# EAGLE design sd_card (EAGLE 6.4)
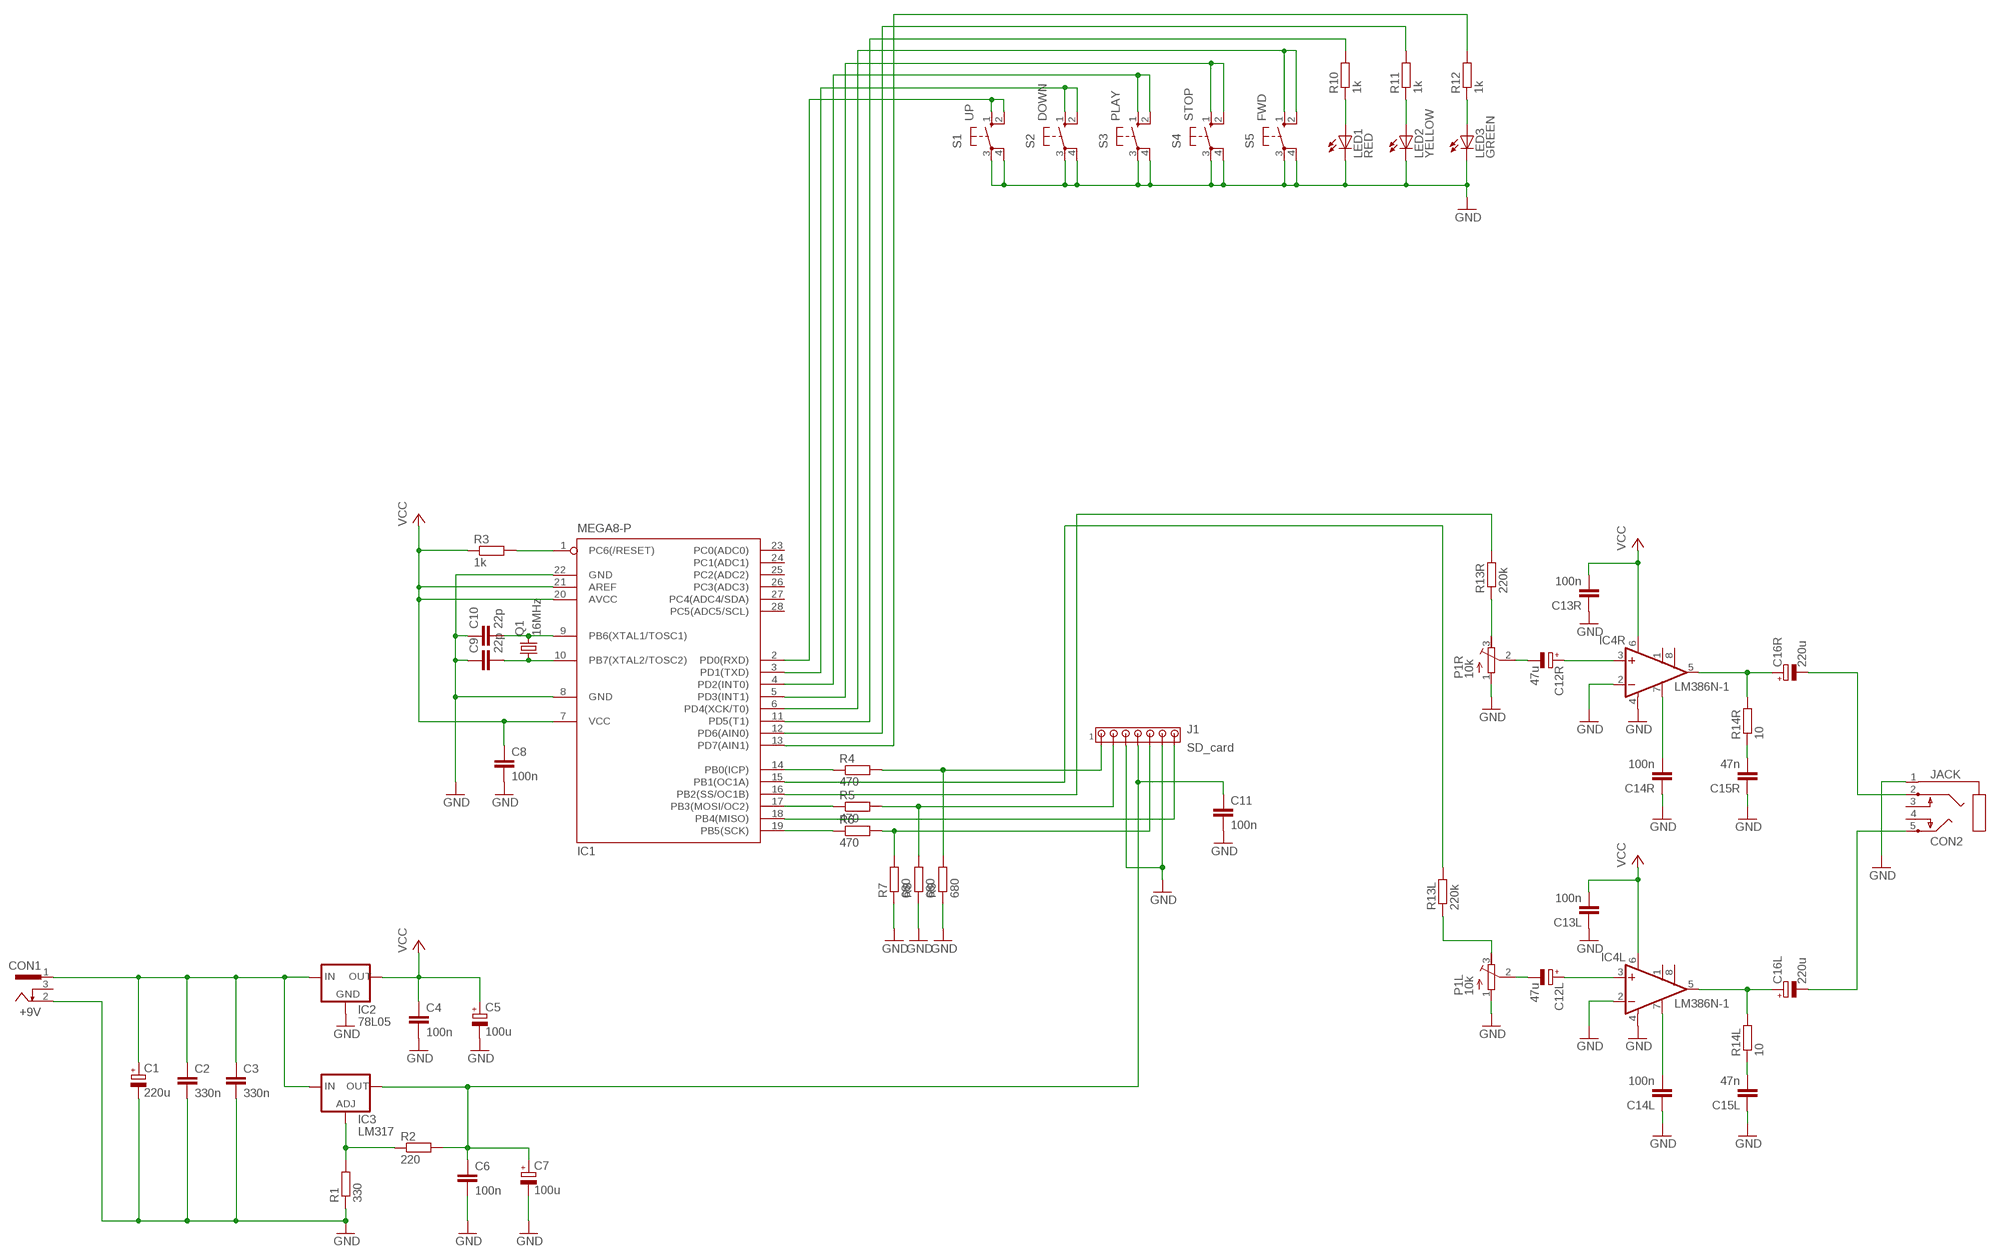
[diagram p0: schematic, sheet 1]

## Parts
C1  220u  CPOL-EUE5-8.5  [E5-8,5]
C2  330n  C-EU025-025X050  [C025-025X050]
C3  330n  C-EU025-025X050  [C025-025X050]
C4  100n  C-EU025-025X050  [C025-025X050]
C5  100u  CPOL-EUE2.5-5  [E2,5-5]
C6  100n  C-EU025-025X050  [C025-025X050]
C7  100u  CPOL-EUE2.5-5  [E2,5-5]
C8  100n  C-EU025-025X050  [C025-025X050]
C9  22p  C-EU025-025X050  [C025-025X050]
C10  22p  C-EU025-025X050  [C025-025X050]
C11  100n  C-EU025-025X050  [C025-025X050]
C12L  47u  CPOL-EUE2.5-5  [E2,5-5]
C12R  47u  CPOL-EUE2.5-5  [E2,5-5]
C13L  100n  C-EU025-025X050  [C025-025X050]
C13R  100n  C-EU025-025X050  [C025-025X050]
C14L  100n  C-EU025-025X050  [C025-025X050]
C14R  100n  C-EU025-025X050  [C025-025X050]
C15L  47n  C-EU025-025X050  [C025-025X050]
C15R  47n  C-EU025-025X050  [C025-025X050]
C16L  220u  CPOL-EUE5-4  [E5-4]
C16R  220u  CPOL-EUE5-4  [E5-4]
CON1  +9V  733980-62  [733980-62]
CON2  JACK  [JACK]
IC1  MEGA8-P  [DIL28-3]
IC2  78L05  78XXL  [78XXL]
IC3  LM317  LM317TL  [317TL]
IC4L  LM386N-1  [DIL08]
IC4R  LM386N-1  [DIL08]
J1  SD_card  MTA07-100  [10X07MTA]
LED1  RED  LED5MM  [LED5MM]
LED2  YELLOW  LED5MM  [LED5MM]
LED3  GREEN  LED5MM  [LED5MM]
P1L  10k  TRIM  [TRIM]
P1R  10k  TRIM  [TRIM]
Q1  16MHz  CRYSTALHC49S  [HC49/S]
R1  330  R-EU_0207/10  [0207/10]
R2  220  R-EU_0207/2V  [0207/2V]
R3  1k  R-EU_0207/10  [0207/10]
R4  470  R-EU_0207/10  [0207/10]
R5  470  R-EU_0207/10  [0207/10]
R6  470  R-EU_0207/10  [0207/10]
R7  680  R-EU_0207/10  [0207/10]
R8  680  R-EU_0207/10  [0207/10]
R9  680  R-EU_0207/10  [0207/10]
R10  1k  R-EU_0207/10  [0207/10]
R11  1k  R-EU_0207/10  [0207/10]
R12  1k  R-EU_0207/10  [0207/10]
R13L  220k  R-EU_0207/2V  [0207/2V]
R13R  220k  R-EU_0207/2V  [0207/2V]
R14L  10  R-EU_0207/10  [0207/10]
R14R  10  R-EU_0207/10  [0207/10]
S1  UP  10-XX  [B3F-10XX]
S2  DOWN  10-XX  [B3F-10XX]
S3  PLAY  10-XX  [B3F-10XX]
S4  STOP  10-XX  [B3F-10XX]
S5  FWD  10-XX  [B3F-10XX]

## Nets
GND: C1.- C2.2 C3.2 C4.2 C5.- C6.2 C7.- C8.2 C9.1 C10.1 C11.2 C13L.1 C13R.1 C14L.1 C14R.1 C15L.1 C15R.1 CON1.2 CON2.1 IC1.8(GND) IC1.22(GND) IC2.GND IC4L.2(-IN) IC4L.4(GND) IC4R.2(-IN) IC4R.4(GND) J1.3 J1.6 LED1.K(C) LED2.K(C) LED3.K(C) P1L.1 P1R.1 R1.1 R7.1 R8.1 R9.1 S1.3(P) S1.4(P1) S2.3(P) S2.4(P1) S3.3(P) S3.4(P1) S4.3(P) S4.4(P1) S5.3(P) S5.4(P1)
N$1: C1.+ C2.1 C3.1 CON1.1 IC2.IN IC3.3(IN)
N$2: IC3.1(ADJ) R1.2 R2.1
N$3: C6.1 C7.+ C11.1 IC3.2(OUT) J1.4 R2.2
N$4: IC1.14(PB0(ICP)) R4.1
N$5: C10.2 IC1.9(PB6(XTAL1/TOSC1)) Q1.2
N$6: C9.2 IC1.10(PB7(XTAL2/TOSC2)) Q1.1
N$7: IC1.17(PB3(MOSI/OC2)) R5.1
N$8: IC1.1(PC6(/RESET)) R3.2
N$9: C12R.+ IC4R.3(+IN)
N$10: IC1.19(PB5(SCK)) R6.1
N$11: J1.5 R6.2 R7.2
N$12: J1.2 R5.2 R8.2
N$13: J1.1 R4.2 R9.2
N$14: IC1.18(PB4(MISO)) J1.7
N$15: C16R.+ IC4R.5(OUT) R14R.2
N$16: C15R.2 R14R.1
N$17: C14R.2 IC4R.7(BYPASS)
N$18: C12R.- P1R.2
N$19: C16L.+ IC4L.5(OUT) R14L.2
N$20: C15L.2 R14L.1
N$21: C14L.2 IC4L.7(BYPASS)
N$22: C12L.+ IC4L.3(+IN)
N$23: LED3.A R12.1
N$24: LED2.A R11.1
N$25: LED1.A R10.1
N$26: IC1.2(PD0(RXD)) S1.1(S) S1.2(S1)
N$27: IC1.3(PD1(TXD)) S2.1(S) S2.2(S1)
N$28: IC1.4(PD2(INT0)) S3.1(S) S3.2(S1)
N$29: IC1.5(PD3(INT1)) S4.1(S) S4.2(S1)
N$30: IC1.6(PD4(XCK/T0)) S5.1(S) S5.2(S1)
N$31: IC1.11(PD5(T1)) R10.2
N$32: IC1.12(PD6(AIN0)) R11.2
N$33: IC1.13(PD7(AIN1)) R12.2
N$69: C12L.- P1L.2
N$70: C16R.- CON2.2
N$71: C16L.- CON2.5
N$73: IC1.16(PB2(SS/OC1B)) R13R.2
N$132: P1R.3 R13R.1
N$133: P1L.3 R13L.1
N$134: IC1.15(PB1(OC1A)) R13L.2
VCC: C4.1 C5.+ C8.1 C13L.2 C13R.2 IC1.7(VCC) IC1.20(AVCC) IC1.21(AREF) IC2.OUT IC4L.6(VS) IC4R.6(VS) R3.1
Unconnected: CON1.3 CON2.3 CON2.4 IC1.23(PC0(ADC0)) IC1.24(PC1(ADC1)) IC1.25(PC2(ADC2)) IC1.26(PC3(ADC3)) IC1.27(PC4(ADC4/SDA)) IC1.28(PC5(ADC5/SCL)) IC4L.1(GAIN) IC4L.8(GAIN) IC4R.1(GAIN) IC4R.8(GAIN)

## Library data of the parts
C1 C5 C7 C12L C12R C16L C16R = resistor:CPOL-EU: POLARIZED CAPACITOR, European symbol
C2-C4 C6 C8-C11 C13L C13R C14L C14R C15L C15R = rcl:C-EU: CAPACITOR, European symbol
CON1 = con-conrad:73398?: FEMALE PRINT CONNECTOR Niedervolt-Steckverbinder Distributor Conrad
CON2 = jack:JACK
IC1 = atmel:MEGA8-P: MICROCONTROLLER 8 Kbytes FLASH, 1 kbytes SRAM, 512 bytes EEPROM, USART, 4-channel 10 bit ADC, 2-channel 8 bit ADC Pin compatible with Atmega48, ATMega88, ATMega168 Source: avr.lbr; OC_FARNELL: unknown; OC_NEWARK: unknown
IC2 = v-reg:78XXL: VOLTAGE REGULATOR
IC3 = v-reg:LM317TL: VOLTAGE REGULATOR
IC4L IC4R = linear:LM386?-*: Low Voltage Audio Power Amplifier Source: http://cache.national.com/ds/LM/LM386.pdf
J1 = con-amp:MTA07-100: AMP connector
LED1-LED3 = led:LED: LED
P1L P1R = trim:TRIM
Q1 = crystal:CRYSTAL: CRYSTAL; OC_FARNELL: 1667008; OC_NEWARK: unknown
R1-R12 R13L R13R R14L R14R = rcl:R-EU_: RESISTOR, European symbol
S1-S5 = switch-omron:10-XX: OMRON SWITCH; MPN: B3F-1000; OC_FARNELL: 176432; OC_NEWARK: 36M3542

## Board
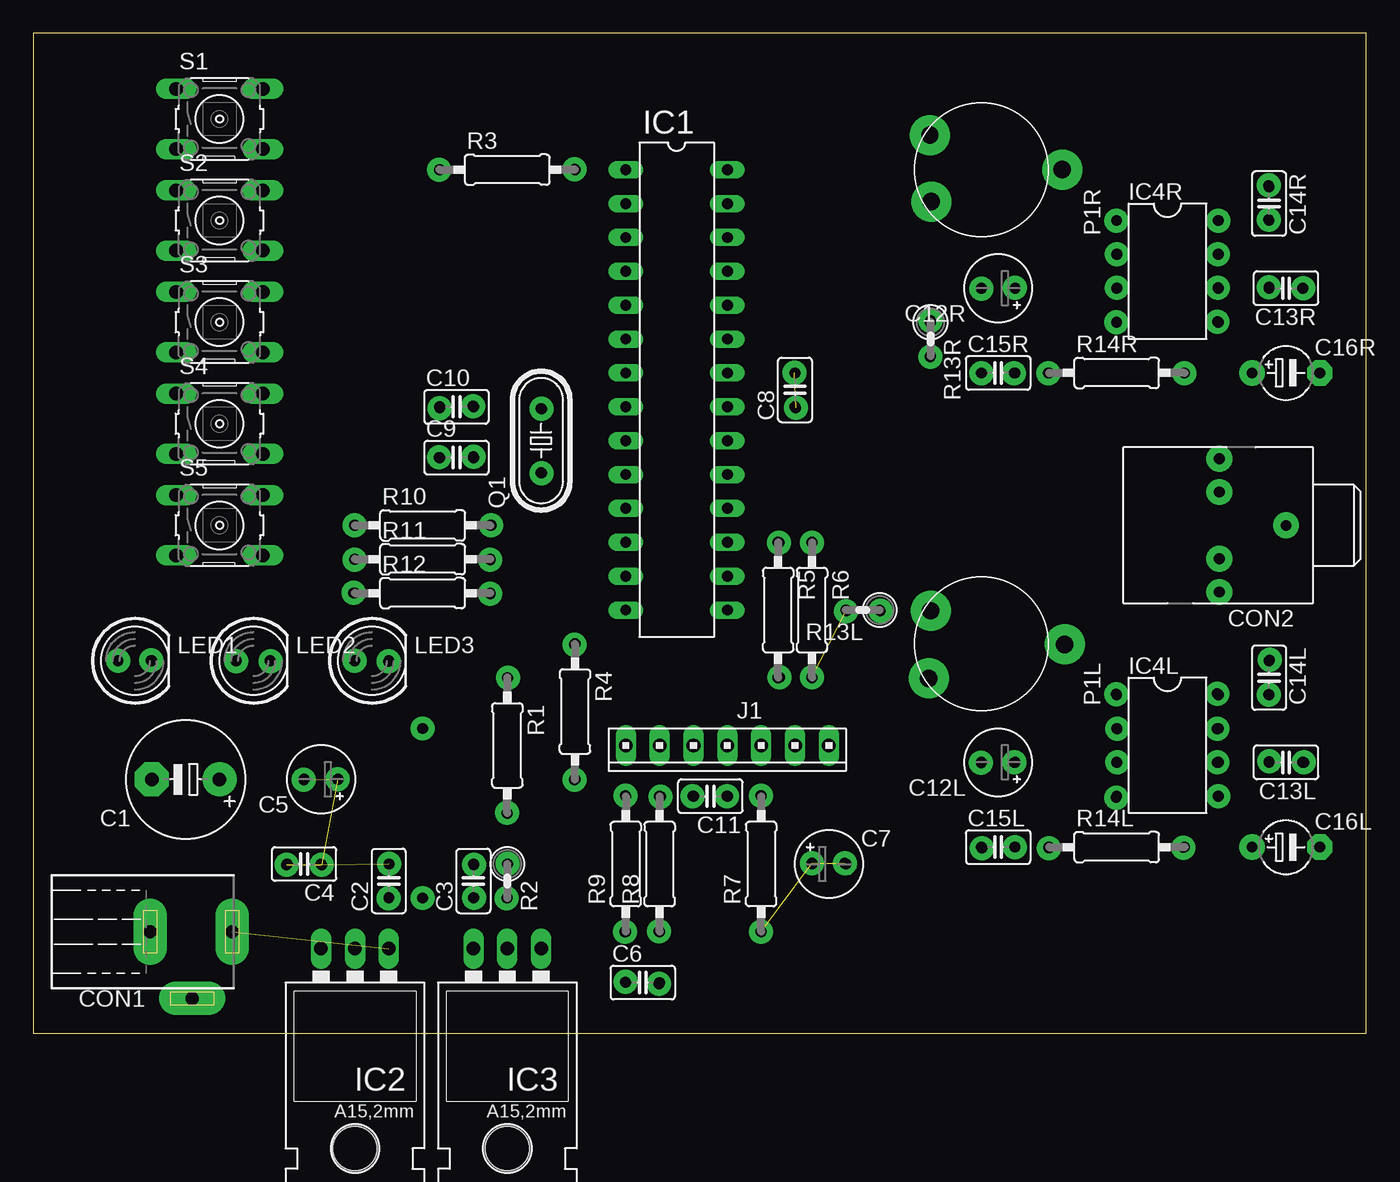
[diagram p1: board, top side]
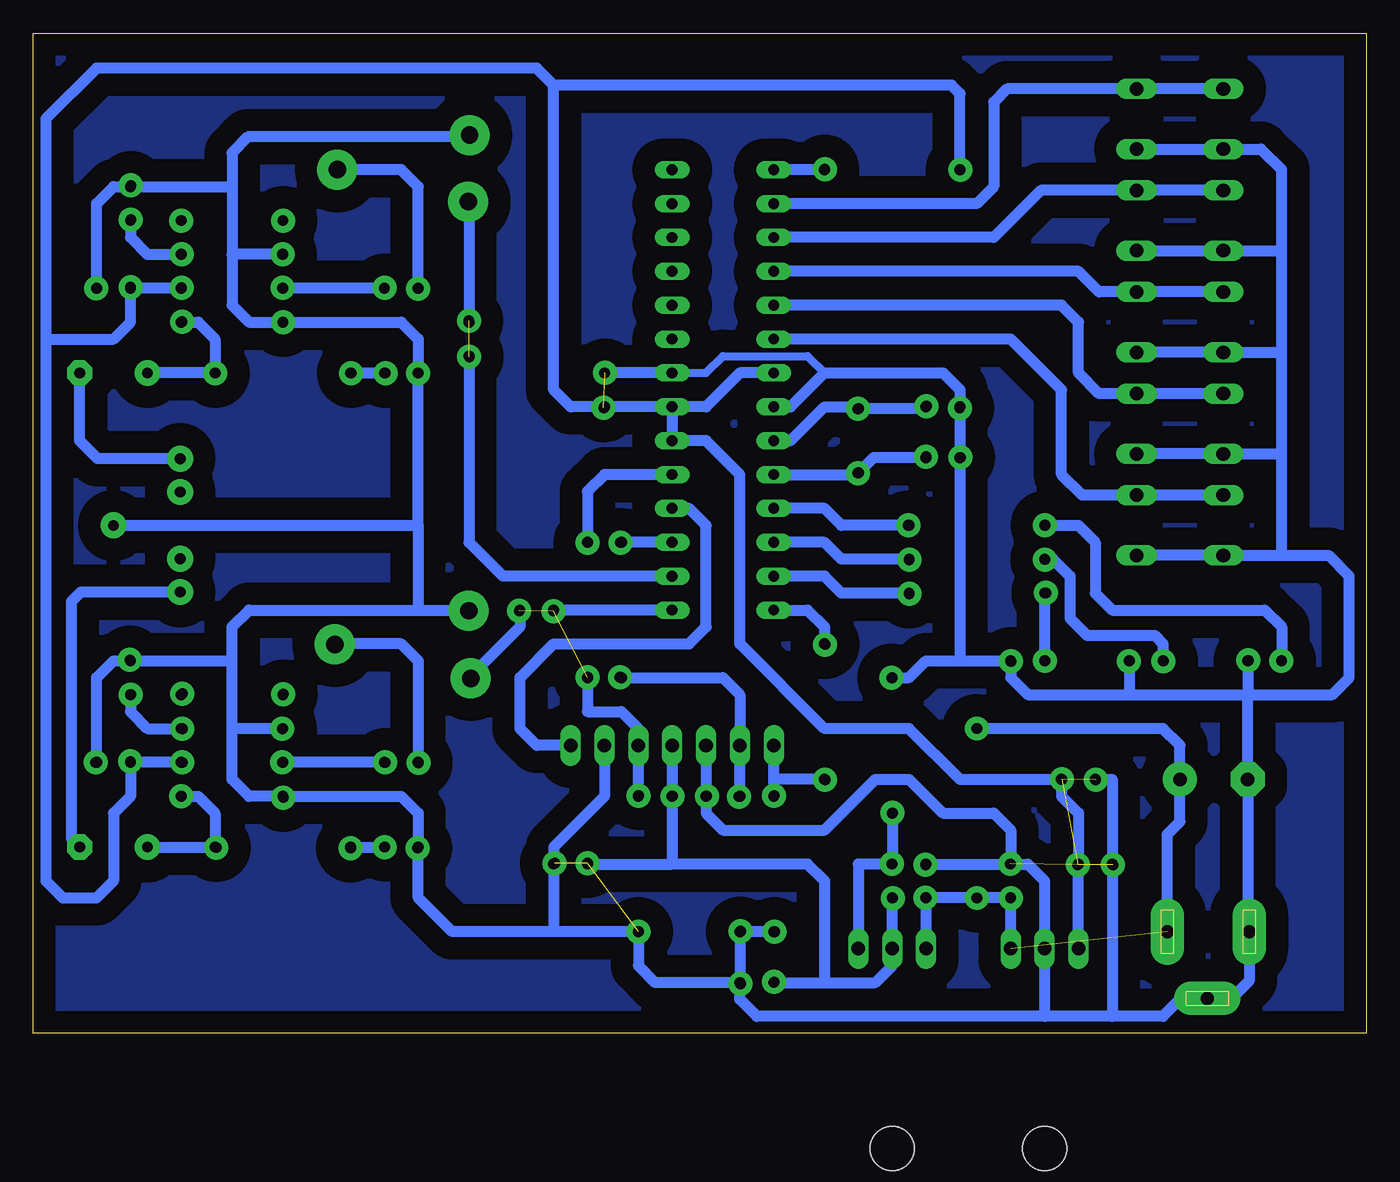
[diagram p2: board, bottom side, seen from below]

Size 100 x 75 mm. Coordinates in mm from the lower left corner, seen from the top.
Outline: 0,0 100,0 100,75 0,75 0,0
Copper layers (1*16): Top 0.035mm / dielectric 1.5mm / Bottom 0.035mm
Design rules "default": minimum track width 10mil, minimum drill 24mil, track to track 8mil, track to pad 8mil, pad to pad 8mil, via to via 8mil, smd to smd 8mil, copper to edge 40mil, drill to drill 8mil, minimum pad ring 10mil, minimum via ring 8mil, stop-mask expansion 4mil, vias tented up to drill 0mil, thermal gap 10mil

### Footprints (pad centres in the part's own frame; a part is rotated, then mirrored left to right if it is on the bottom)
E5-8,5 = drill 1.016 pad 2.54: + -2.54,0 | drill 1.016 pad 2.54 octagon: - 2.54,0
C025-025X050 = drill 0.813 octagon: 1 -1.27,0; 2 1.27,0
E2,5-5 = drill 0.813 pad 1.6: + -1.27,0 | drill 0.813 pad 1.6 octagon: - 1.27,0
E5-4 = drill 0.813 pad 1.905: + -2.54,0 | drill 0.813 pad 1.905 octagon: - 2.54,0
733980-62 = drill 1 pad 2.5 long: 1 0,8.57; 2 0,2.42; 3 5,5.57
JACK = drill 0.8 pad 1.93: 1 -5.08,0; 2 -0.08,-5; 3 -0.08,2.5; 4 -0.08,-2.5; 5 -0.08,5
DIL28-3 = drill 0.813 long: 1 -16.51,-3.81; 2 -13.97,-3.81; 3 -11.43,-3.81; 4 -8.89,-3.81; 5 -6.35,-3.81; 6 -3.81,-3.81; 7 -1.27,-3.81; 8 1.27,-3.81; 9 3.81,-3.81; 10 6.35,-3.81; 11 8.89,-3.81; 12 11.43,-3.81; 13 13.97,-3.81; 14 16.51,-3.81; 15 16.51,3.81; 16 13.97,3.81; 17 11.43,3.81; 18 8.89,3.81; 19 6.35,3.81; 20 3.81,3.81; 21 1.27,3.81; 22 -1.27,3.81; 23 -3.81,3.81; 24 -6.35,3.81; 25 -8.89,3.81; 26 -11.43,3.81; 27 -13.97,3.81; 28 -16.51,3.81
78XXL = drill 1.016 long: GND 0,-3.81; IN -2.54,-3.81; OUT 2.54,-3.81 | hole 3.302: 0,11.176
317TL = drill 1.016 long: 1 -2.54,-3.81; 2 0,-3.81; 3 2.54,-3.81 | hole 3.302: 0,11.176
DIL08 = drill 0.813 pad 1.27: 1 -3.81,-3.81; 2 -1.27,-3.81; 3 1.27,-3.81; 4 3.81,-3.81; 5 3.81,3.81; 6 1.27,3.81; 7 -1.27,3.81; 8 -3.81,3.81
10X07MTA = drill 1.016 long: 1 7.62,0; 2 5.08,0; 3 2.54,0; 4 0,0; 5 -2.54,0; 6 -5.08,0; 7 -7.62,0
LED5MM = drill 0.813 octagon: A -1.27,0; K 1.27,0
TRIM = drill 0.61 pad 1.778: 1 -2.46,-3.81; 2 0,6.19; 3 2.54,-3.81
HC49/S = drill 0.813: 1 -2.413,0; 2 2.413,0
0207/10 = drill 0.813 octagon: 1 -5.08,0; 2 5.08,0
0207/2V = drill 0.813 octagon: 1 -1.27,0; 2 1.27,0
B3F-10XX = drill 1.016 long: 1 -3.251,2.261; 2 3.251,2.261; 3 -3.251,-2.261; 4 3.251,-2.261

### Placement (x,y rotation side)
C1  11.43,19.05 180 top
C2  26.67,11.43 90 top
C3  33.02,11.43 90 top
C4  20.32,12.7 180 top
C5  21.59,19.05 180 top
C6  45.72,3.81 0 top
C7  59.69,12.7 0 top
C8  57.15,48.26 90 top
C9  31.75,43.18 0 top
C10  31.75,46.99 0 top
C11  50.8,17.78 180 top
C12L  72.39,20.32 180 top
C12R  72.39,55.88 180 top
C13L  93.98,20.32 180 top
C13R  93.98,55.88 180 top
C14L  92.71,26.67 270 top
C14R  92.71,62.23 270 top
C15L  72.39,13.97 0 top
C15R  72.39,49.53 0 top
C16L  93.98,13.97 0 top
C16R  93.98,49.53 0 top
CON1  6.35,7.62 270 top
CON2  88.9,38.1 180 top
IC1  48.26,48.26 270 top
IC2  24.13,2.54 180 top
IC3  35.56,2.54 180 top
IC4L  85.09,21.59 270 top
IC4R  85.09,57.15 270 top
J1  52.07,21.59 180 top
LED1  7.62,27.94 0 top
LED2  16.51,27.94 0 top
LED3  25.4,27.94 0 top
P1L  71.12,29.21 270 top
P1R  71.12,64.77 270 top
Q1  38.1,44.45 90 top
R1  35.56,21.59 270 top
R2  35.56,11.43 270 top
R3  35.56,64.77 0 top
R4  40.64,24.13 270 top
R5  55.88,31.75 270 top
R6  58.42,31.75 270 top
R7  54.61,12.7 90 top
R8  46.99,12.7 90 top
R9  44.45,12.7 90 top
R10  29.21,38.1 0 top
R11  29.21,35.56 0 top
R12  29.21,33.02 0 top
R13L  62.23,31.75 180 top
R13R  67.31,52.07 270 top
R14L  81.28,13.97 0 top
R14R  81.28,49.53 0 top
S1  13.97,68.58 0 top
S2  13.97,60.96 0 top
S3  13.97,53.34 0 top
S4  13.97,45.72 0 top
S5  13.97,38.1 0 top

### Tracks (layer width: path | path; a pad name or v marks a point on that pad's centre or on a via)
GND
  Bottom 0.61: IC1.22 49.53,49.53 48.26,50.8 41.91,50.8 40.64,49.53
  Bottom 0.813: 19.05,1.27 C4.2 19.05,19.05 C5.- | 24.13,1.27 IC2.GND 24.13,11.43 25.4,12.7 C2.2 | C3.2 C2.2 | 19.05,1.27 15.24,1.27 13.97,2.54 10.16,2.54 8.77,3.93 CON1.2 8.89,7.74 C1.- 8.89,25.4 | 19.05,1.27 24.13,1.27 | 24.13,1.27 45.72,1.27 46.99,2.54 C6.2 | R9.1 R8.1 C6.2 | P1R.1 83.9,67.23 85.09,66.04 85.09,63.5 | 85.09,63.5 85.09,58.42 | 85.09,58.42 85.09,54.61 83.82,53.34 IC4R.4 72.39,53.34 71.12,52.07 C15R.1 71.12,38.1 | IC4R.2 85.09,58.42 | 85.09,63.5 C14R.1 93.98,63.5 95.25,62.23 C13R.1 | 85.09,22.86 85.09,19.05 83.82,17.78 IC4L.4 72.39,17.78 71.12,16.51 C15L.1 71.12,10.16 68.58,7.62 60.96,7.62 | 85.09,22.86 85.09,27.94 | 85.09,27.94 85.09,30.48 83.82,31.75 71.12,31.75 | 71.12,31.75 67.39,31.75 P1L.1 | IC4L.2 85.09,22.86 | 85.09,27.94 C14L.1 93.98,27.94 95.25,26.67 C13L.1 | CON2.1 71.12,38.1 | 71.12,38.1 71.12,31.75 | 6.35,35.84 6.35,43.18 | 6.35,43.18 6.35,50.8 | 6.35,50.8 6.35,58.42 | 6.35,58.42 6.35,64.77 7.9,66.32 S1.3 S1.4 | S2.4 S2.3 6.63,58.7 6.35,58.42 | 6.35,50.8 6.63,51.08 S3.3 S3.4 | S5.4 S5.3 6.35,35.84 | IC1.8 43.18,46.99 40.64,49.53 31.75,49.53 30.48,48.26 C10.1 C9.1 30.48,27.94 | 17.78,25.4 25.4,25.4 26.67,26.67 LED3.K 30.48,27.94 | 17.78,25.4 8.89,25.4 | 8.89,25.4 2.54,25.4 1.27,26.67 1.27,34.29 2.82,35.84 6.35,35.84 | 6.35,43.18 6.63,43.46 S4.3 S4.4 | LED1.K 8.89,25.4 | LED2.K 17.78,25.4 | IC1.22 C8.2 | J1.3 C11.2 49.53,16.51 48.26,15.24 40.64,15.24 36.83,19.05 34.29,19.05 31.75,16.51 27.94,16.51 26.67,15.24 C2.2 | 60.96,7.62 R7.1 54.61,5.08 53.34,3.81 C6.2 | R1.1 34.29,26.67 33.02,27.94 30.48,27.94 | J1.6 57.15,17.78 60.96,13.97 C7.- 60.96,7.62
N$1  (via drill 0.8 pad 1.78)  (1 unrouted)
  Bottom 0.813: IC2.IN C2.1 v29.21,10.16 C3.1 IC3.3 | 29.21,22.86 15.24,22.86 13.97,21.59 13.97,19.68 C1.+ 13.97,15.88 14.92,14.93 CON1.1
N$2
  Bottom 0.813: IC3.1 38.1,12.7 R2.1 R1.2
N$3
  Bottom 0.813: R2.2 IC3.2 35.56,5.08 36.83,3.81 40.64,3.81 | 52.07,12.7 41.91,12.7 40.64,11.43 40.64,3.81 | C6.1 40.64,3.81 | J1.4 C11.1 52.07,12.7 | C7.+ 52.07,12.7
N$4
  Bottom 0.813: IC1.14 41.91,31.75 40.64,30.48 R4.1
N$5
  Bottom 0.813: IC1.9 43.18,44.45 40.64,46.99 38.23,46.99 Q1.2 33.15,46.86 C10.2
N$6
  Bottom 0.813: IC1.10 38.23,41.91 Q1.1 36.96,43.18 C9.2
N$7
  Bottom 0.813: IC1.17 R5.1
N$8
  Bottom 0.813: R3.2 IC1.1
N$9
  Bottom 0.813: C12R.+ IC4R.3
N$10
  Bottom 0.813: IC1.19 57.15,41.91 58.42,40.64 R6.1
N$11
  Bottom 0.813: R7.2 J1.5 54.61,22.86 55.88,24.13 58.42,24.13 R6.2
N$12
  Bottom 0.813: R8.2 J1.2 46.99,25.4 48.26,26.67 R5.2
N$13
  Bottom 0.813: R9.2 44.45,19.05 | 44.45,19.05 J1.1 | R4.2 44.45,19.05
N$14
  Bottom 0.813: J1.7 62.23,21.59 63.5,22.86 63.5,26.67 60.96,29.21 50.8,29.21 49.53,30.48 49.53,38.1 50.8,39.37 IC1.18
N$15
  Bottom 0.813: C16R.+ R14R.2 86.36,52.07 87.63,53.34 IC4R.5
N$16
  Bottom 0.813: R14R.1 C15R.2
N$17
  Bottom 0.813: C14R.2 92.71,59.69 91.44,58.42 IC4R.7
N$18
  Bottom 0.813: C12R.- 71.12,63.5 72.39,64.77 P1R.2
N$19
  Bottom 0.813: C16L.+ R14L.2 86.36,16.51 87.63,17.78 IC4L.5
N$20
  Bottom 0.813: R14L.1 C15L.2
N$21
  Bottom 0.813: C14L.2 92.71,24.13 91.44,22.86 IC4L.7
N$22
  Bottom 0.813: C12L.+ IC4L.3
N$23
  Bottom 0.813: R12.1 LED3.A
N$24
  Bottom 0.813: R11.1 23.5,35.56 22.23,34.29 22.23,31.11 20.95,29.84 15.88,29.84 15.24,29.21 LED2.A
N$25
  Bottom 0.813: R10.1 21.59,38.1 20.32,36.83 20.32,33.02 19.05,31.75 7.62,31.75 6.35,30.48 LED1.A
N$26
  Bottom 0.813: S1.1 S1.2 26.95,70.84 27.94,69.85 27.94,63.5 29.21,62.23 IC1.2
N$27
  Bottom 0.813: S2.1 S2.2 24.41,63.22 27.94,59.69 IC1.3
N$28
  Bottom 0.813: S3.1 S3.2 20.04,55.6 21.59,57.15 IC1.4
N$29
  Bottom 0.813: S4.1 S4.2 20.04,47.98 21.59,49.53 21.59,53.34 22.86,54.61 IC1.5
N$30
  Bottom 0.813: S5.1 S5.2 21.31,40.36 22.86,41.91 22.86,48.26 26.67,52.07 IC1.6
N$31
  Bottom 0.813: R10.2 39.37,38.1 40.64,39.37 IC1.11
N$32
  Bottom 0.813: R11.2 39.37,35.56 40.64,36.83 IC1.12
N$33
  Bottom 0.813: R12.2 39.37,33.02 40.64,34.29 IC1.13
N$35  (via drill 0.8 pad 1.78)
  other vias: 29.21,22.86
N$36  (via drill 0.8 pad 1.8)
  other vias: 26.67,10.14
N$37  (via drill 0.8 pad 1.8)  (4 unrouted)
  other vias: 26.71,12.7 21.64,12.63 18.99,12.63 20.3,19.01 22.82,19.04
N$38  (via drill 0.8 pad 1.8)
  other vias: 35.6,26.65
N$39  (via drill 0.8 pad 1.8)
  other vias: 35.55,16.53
N$40  (via drill 0.8 pad 1.8)
  other vias: 35.59,12.7
N$41  (via drill 0.8 pad 1.8)
  other vias: 35.51,10.14
N$42  (via drill 0.8 pad 1.8)
  other vias: 33.06,10.18
N$43  (via drill 0.8 pad 1.8)
  other vias: 33.06,12.63
N$44
  pour Bottom (isolate 1.676): 0,74.93 100.33,74.93 100.33,0 0,0
N$46  (via drill 0.8 pad 1.8)
  other vias: 40.59,19.02
N$47  (via drill 0.8 pad 1.8)
  other vias: 44.42,17.83
N$48  (via drill 0.8 pad 1.8)
  other vias: 47.05,17.76
N$49  (via drill 0.8 pad 1.8)
  other vias: 49.47,17.79
N$50  (via drill 0.8 pad 1.8)
  other vias: 52.03,17.79
N$51  (via drill 0.8 pad 1.8)
  other vias: 54.59,17.83
N$52  (via drill 0.8 pad 1.8)  (2 unrouted)
  other vias: 60.89,12.76 58.42,12.76 54.59,7.64
N$53  (via drill 0.8 pad 1.8)
  other vias: 44.38,7.61
N$54  (via drill 0.8 pad 1.8)
  other vias: 46.94,7.65
N$55  (via drill 0.8 pad 1.8)
  other vias: 46.94,3.72
N$56  (via drill 0.8 pad 1.8)
  other vias: 44.42,3.86
N$57  (via drill 0.8 pad 1.8)
  other vias: 6.36,27.94
N$58  (via drill 0.8 pad 1.8)
  other vias: 8.84,27.97
N$59  (via drill 0.8 pad 1.8)
  other vias: 15.21,27.92
N$60  (via drill 0.8 pad 1.8)
  other vias: 17.79,27.92
N$61  (via drill 0.8 pad 1.8)
  other vias: 24.1,27.94
N$62  (via drill 0.8 pad 1.8)
  other vias: 26.66,27.89
N$63  (via drill 0.8 pad 1.8)
  other vias: 24.09,38.1
N$64  (via drill 0.8 pad 1.8)
  other vias: 24.11,35.53
N$65  (via drill 0.8 pad 1.8)
  other vias: 24.03,33.03
N$66  (via drill 0.8 pad 1.8)
  other vias: 34.36,38.1
N$67  (via drill 0.8 pad 1.8)
  other vias: 34.28,35.51
N$68  (via drill 0.8 pad 1.8)
  other vias: 34.28,32.97
N$69
  Bottom 0.813: P1L.2 72.39,29.21 71.12,27.94 C12L.-
N$70
  Bottom 0.813: C16R.- 96.52,44.45 95.17,43.1 CON2.2
N$71
  Bottom 0.813: C16L.- 97.16,14.61 97.16,32.38 96.44,33.1 CON2.5
N$73
  Bottom 0.813: IC1.16 64.77,34.29 67.31,36.83 R13R.2
N$74  (via drill 0.8 pad 1.8)
  other vias: 38.13,46.83
N$75  (via drill 0.8 pad 1.8)
  other vias: 38.13,42.02
N$76  (via drill 0.8 pad 1.8)
  other vias: 30.49,46.89
N$77  (via drill 0.8 pad 1.8)
  other vias: 32.99,47.04
N$78  (via drill 0.8 pad 1.8)
  other vias: 33.02,43.25
N$79  (via drill 0.8 pad 1.8)
  other vias: 30.43,43.19
N$80  (via drill 0.8 pad 1.8)  (1 unrouted)
  other vias: 57.11,49.53 57.2,46.91
N$81  (via drill 0.8 pad 1.8)  (1 unrouted)
  other vias: 67.32,53.45 67.29,50.75
N$82  (via drill 0.8 pad 1.8)
  other vias: 30.46,64.76
N$83  (via drill 0.8 pad 1.8)
  other vias: 40.62,64.8
N$84  (via drill 0.8 pad 1.8)
  other vias: 40.59,29.16
N$85  (via drill 0.8 pad 1.8)
  other vias: 55.95,36.81
N$86  (via drill 0.8 pad 1.8)
  other vias: 58.4,36.81
N$87  (via drill 0.8 pad 1.8)  (2 unrouted)
  other vias: 58.4,26.71 60.99,31.67 63.54,31.69
N$88  (via drill 0.8 pad 1.8)
  other vias: 55.99,26.71
N$89  (via drill 0.8 pad 1.8)
  other vias: 81.24,25.44
N$90  (via drill 0.8 pad 1.8)
  other vias: 81.32,22.84
N$91  (via drill 0.8 pad 1.8)
  other vias: 81.32,20.32
N$92  (via drill 0.8 pad 1.8)
  other vias: 81.24,17.68
N$93  (via drill 0.8 pad 1.8)
  other vias: 71.17,13.89
N$94  (via drill 0.8 pad 1.8)
  other vias: 76.19,13.89
N$95  (via drill 0.8 pad 1.8)
  other vias: 73.63,13.97
N$96  (via drill 0.8 pad 1.8)
  other vias: 88.82,25.48
N$97  (via drill 0.8 pad 1.8)
  other vias: 88.82,22.84
N$98  (via drill 0.8 pad 1.8)
  other vias: 88.82,20.32
N$99  (via drill 0.8 pad 1.8)
  other vias: 88.9,17.79
N$100  (via drill 0.8 pad 1.8)
  other vias: 86.28,13.93
N$101  (via drill 0.8 pad 1.8)
  other vias: 92.72,20.39
N$102  (via drill 0.8 pad 1.8)
  other vias: 95.32,20.32
N$103  (via drill 0.8 pad 1.8)
  other vias: 92.69,25.41
N$104  (via drill 0.8 pad 1.8)
  other vias: 92.76,28
N$105  (via drill 0.8 pad 1.8)
  other vias: 81.27,60.95
N$106  (via drill 0.8 pad 1.8)
  other vias: 81.31,58.43
N$107  (via drill 0.8 pad 1.8)
  other vias: 81.31,55.9
N$108  (via drill 0.8 pad 1.8)
  other vias: 81.27,53.34
N$109  (via drill 0.8 pad 1.8)
  other vias: 73.58,49.51
N$110  (via drill 0.8 pad 1.8)
  other vias: 76.15,49.51
N$111  (via drill 0.8 pad 1.8)
  other vias: 71.12,49.51
N$112  (via drill 0.8 pad 1.8)
  other vias: 86.35,49.51
N$113  (via drill 0.8 pad 1.8)
  other vias: 88.85,53.37
N$114  (via drill 0.8 pad 1.8)
  other vias: 88.89,55.94
N$115  (via drill 0.8 pad 1.8)
  other vias: 88.89,58.43
N$116  (via drill 0.8 pad 1.8)
  other vias: 88.92,60.95
N$117  (via drill 0.8 pad 1.8)
  other vias: 92.68,63.59
N$118  (via drill 0.8 pad 1.8)
  other vias: 92.68,61.03
N$119  (via drill 0.8 pad 1.8)
  other vias: 92.71,55.97
N$120  (via drill 0.8 pad 1.8)
  other vias: 95.27,55.87
N$121  (via drill 0.8 pad 1.8)
  other vias: 71.13,55.86
N$122  (via drill 0.8 pad 1.8)
  other vias: 73.66,55.91
N$123  (via drill 0.8 pad 1.8)
  other vias: 71.11,20.3
N$124  (via drill 0.8 pad 1.8)
  other vias: 73.61,20.32
N$125  (via drill 1.3 pad 3)
  other vias: 67.26,67.37
N$126  (via drill 1.3 pad 3)
  other vias: 67.37,62.38
N$127  (via drill 1.3 pad 3)
  other vias: 77.19,64.78
N$128  (via drill 1.3 pad 3)
  other vias: 67.33,31.7
N$129  (via drill 1.3 pad 3)
  other vias: 67.18,26.62
N$130  (via drill 1.3 pad 3)
  other vias: 77.38,29.17
N$132
  Bottom 0.813: P1R.3 R13R.1
N$133
  Bottom 0.813: R13L.1 63.5,30.48 P1L.3
N$134
  Bottom 0.813: IC1.15 R13L.2
VCC
  Bottom 0.813: IC2.OUT C4.1 21.59,16.51 22.86,17.78 C5.+ 30.48,19.05 34.29,22.86 40.64,22.86 46.99,29.21 46.99,41.91 49.53,44.45 IC1.20 IC1.21 | IC4R.6 C13R.2 92.71,53.34 93.98,52.07 99.06,52.07 | IC4L.6 C13L.2 92.71,17.78 93.98,16.51 93.98,11.43 95.25,10.16 97.79,10.16 99.06,11.43 99.06,52.07 | IC1.21 C8.1 59.69,46.99 60.96,48.26 60.96,71.12 | 60.96,71.12 62.23,72.39 95.25,72.39 99.06,68.58 99.06,52.07 | R3.1 30.48,70.48 31.11,71.12 60.96,71.12 | IC1.7 46.99,49.53 49.53,46.99 IC1.21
